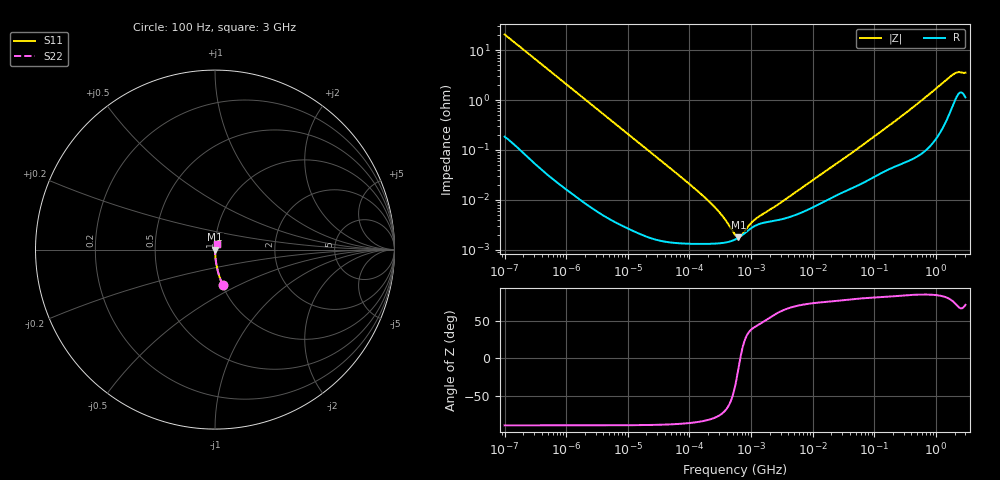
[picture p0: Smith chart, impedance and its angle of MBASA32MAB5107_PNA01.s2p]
! MBASA32MAB5107_PNA01  S-PARAMETER MODEL  ( Standard Model )
! Model Generated by TAIYO YUDEN Corporation (http://www.ty-top.com)
! Version 1.0
! TAIYO YUDEN Control No. 220601
! Copyright(c) 2021 TAIYO YUDEN CO.,LTD. All Rights Reserved.
! Product Description (link to TY-COMPAS)
! https://ds.yuden.co.jp/TYCOMPAS/or/detail?pn=MBASA32MAB5107MPNA01&u=M
! Products Name : Multilayer Ceramic Capacitors
! Characteristics :
!  Capacitance : 100 [uF] , Rated Voltage : 4 [V] , TCC : X5R
!  Case Size : 3.2 x 2.5 / 0.126 x 0.098 [mm/inch] , Thickness : 2.5 / 0.098 [mm/inch]
!  (Conditions: Temperature = 25 [degC] , DC Bias Voltage = 0 [V])
! External Node Assignments :
!  1  o---| |---o  2
! GND o---------o GND
! Frequency Range : 100Hz  -  3GHz  [ 401 STEP ]
# MHZ S RI R 50
! Freq[MHz].  S11 Real  S11 Imag  S21 Real  S21 Imag  S12 Real  S12 Imag  S22 Real  S22 Imag
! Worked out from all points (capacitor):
!   401 points, 100 Hz to 3 GHz, reference 50 ohm
!   read as one part in series: C = 77.3 uF near 109 Hz
!   lowest |Z| = 1.8 mohm at 623.2 kHz (marker M1)
!   series resonance near 667.2 kHz, so ESL is about 740 pH
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0.0001  0.0422 -0.1965  0.9578 0.1965  0.9578 0.1965  0.0422 -0.1965
0.000114  0.0331 -0.1745  0.9669 0.1745  0.9669 0.1745  0.0331 -0.1745
0.000175  0.0147 -0.1161  0.9853 0.1161  0.9853 0.1161  0.0147 -0.1161
0.000348  0.00398 -0.0592  0.996 0.0592  0.996 0.0592  0.00398 -0.0592
0.000724  0.00104 -0.0286  0.999 0.0286  0.999 0.0286  0.00104 -0.0286
0.001788  0.000231 -0.0117  0.9998 0.0117  0.9998 0.0117  0.000231 -0.0117
0.031977  1.58e-05 -0.000659  1 0.000659  1 0.000659  1.58e-05 -0.000659
0.178874  1.32e-05 -0.00011  1 0.00011  1 0.00011  1.32e-05 -0.00011
0.194955  1.32e-05 -9.95e-05  1 9.95e-05  1 9.95e-05  1.32e-05 -9.95e-05
0.21248  1.32e-05 -8.98e-05  1 8.98e-05  1 8.98e-05  1.32e-05 -8.98e-05
0.547723  1.6e-05 -1.24e-05  1 1.24e-05  1 1.24e-05  1.6e-05 -1.24e-05
0.623217  1.75e-05 -4.18e-06  1 4.18e-06  1 4.18e-06  1.75e-05 -4.18e-06
3.339322  4.18e-05 8.66e-05  1 -8.66e-05  1 -8.66e-05  4.18e-05 8.66e-05
3.79959  4.37e-05 9.83e-05  1 -9.83e-05  1 -9.83e-05  4.37e-05 9.83e-05
9.794414  6.99e-05 0.000235  0.9999 -0.000235  0.9999 -0.000235  6.99e-05 0.000235
40.53601  0.000166 0.000813  0.9998 -0.000813  0.9998 -0.000813  0.000166 0.000813
175.1444  0.000424 0.00308  0.9996 -0.00308  0.9996 -0.00308  0.000424 0.00308
471.3361  0.000773 0.0079  0.9992 -0.0079  0.9992 -0.0079  0.000773 0.0079
1868.531  0.00853 0.0307  0.9915 -0.0307  0.9915 -0.0307  0.00853 0.0307
2126.076  0.012 0.0327  0.988 -0.0327  0.988 -0.0327  0.012 0.0327
2317.205  0.0142 0.0328  0.9858 -0.0328  0.9858 -0.0328  0.0142 0.0328
3000  0.0122 0.0326  0.9878 -0.0326  0.9878 -0.0326  0.0122 0.0326
